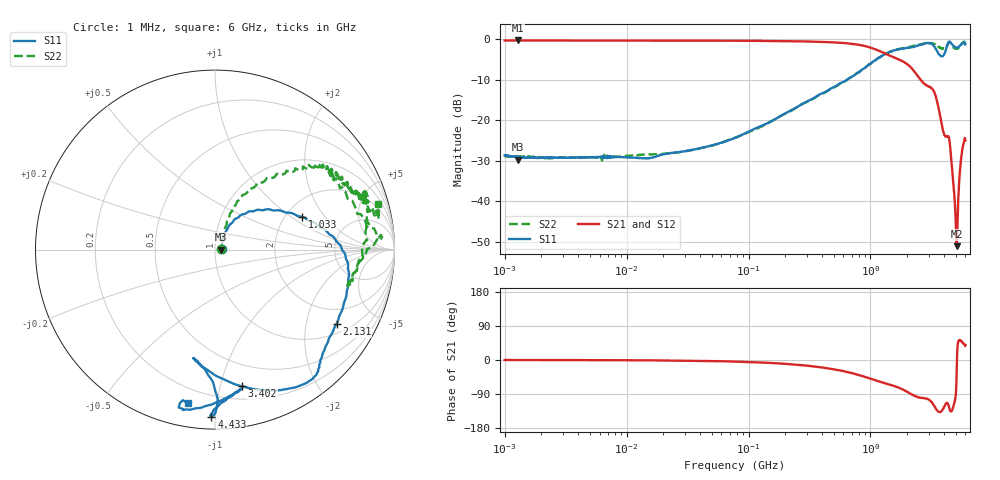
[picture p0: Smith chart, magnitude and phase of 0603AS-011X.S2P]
!s-Parameter Generated by FASTRON Sdn. Bhd.
!FASTRON P/N : 0603AS-011X
!Keysight Technologies: E5071C_MY46733604_B.14.02
!Date: Thu Nov 23 09:53:46 2023
!Version  :Rev01  Thu Nov 23 09:53:46 2023
!Data & Calibration Information:
!Freq  S11:SOLT2(ON)  S21:SOLT2(ON)  S12:SOLT2(ON)  S22:SOLT2(ON)
!PortZ  Port1:50+j0  Port2:50+j0
!When reading reference impedance value at option line is always used.
! Remarks : This data is being provided solely for informational purposes.
# Hz S dB R 50
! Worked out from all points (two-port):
!   1601 points, 1 MHz to 6 GHz, reference 50 ohm
!   highest |S21| = -0.29 dB at 1.281 MHz (marker M1); lowest = -51.1 dB at 5.105 GHz (marker M2)
!   |S21| within 3 dB of the highest: start of sweep to 1.274 GHz
!   lowest |S11| = -29.7 dB at 1.288 MHz (marker M3), VSWR 1.07, Z = 53.4 + j0.0425 ohm
!   |S11| at or under -10 dB: start of sweep to 641.8 MHz
!   |S22| runs from -30.0 to -0.5 dB; largest |S21 - S12| = 0.0099
!   S11 on the Smith chart (normalised r, x): 1 MHz: 1.08, +0.00; 1.033 GHz: 2.45, +1.22; 2.131 GHz: 1.35, -3.01; 3.402 GHz: 0.30, -1.17; 4.433 GHz: 0.07, -0.98; 6 GHz: 0.12, -0.83
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1000000  -28.66 3.2  -0.31 -0.0  -0.31 -0.1  -28.85 2.9
1281258  -28.89 3.6  -0.29 -0.1  -0.31 -0.1  -29.15 -1.2
1287650  -29.70 0.7  -0.33 0.0  -0.30 -0.0  -28.61 0.9
4277066  -29.22 4.9  -0.32 -0.3  -0.31 -0.3  -29.21 5.1
1.823719e7  -28.75 16.4  -0.32 -1.0  -0.33 -1.0  -28.36 18.0
7.757876e7  -24.37 46.8  -0.36 -4.1  -0.36 -4.1  -24.32 48.1
3.307917e8  -14.77 57.3  -0.57 -16.4  -0.57 -16.4  -14.92 66.8
6.136873e8  -10.39 44.8  -0.94 -30.1  -0.94 -30.1  -10.45 64.8
1.032581e9  -5.71 20.6  -2.20 -50.8  -2.21 -50.8  -5.66 50.8
1.414819e9  -3.22 2.8  -3.94 -64.7  -3.94 -64.7  -3.25 41.1
2.130642e9  -2.01 -31.4  -6.91 -89.0  -6.92 -88.9  -1.78 29.9
2.98045e9  -0.90 -53.5  -11.67 -104.0  -11.64 -103.9  -0.93 19.4
3.401721e9  -2.19 -78.7  -13.72 -125.7  -13.71 -125.8  -1.34 9.1
3.644712e9  -3.69 -96.3  -17.57 -137.3  -17.57 -137.4  -1.92 -8.4
3.887702e9  -4.21 -100.9  -21.87 -131.7  -21.87 -131.8  -2.28 -14.1
4.433128e9  -0.60 -91.2  -24.95 -127.3  -24.98 -127.3  -0.60 4.2
4.656967e9  -1.23 -88.5  -31.64 -132.8  -31.67 -132.8  -1.57 13.7
4.936766e9  -1.94 -80.4  -41.33 -105.1  -41.37 -105.0  -2.15 30.4
5.104645e9  -2.05 -79.4  -51.11 -10.7  -51.24 -10.9  -2.28 32.7
5.244544e9  -1.99 -80.4  -39.53 48.4  -39.59 48.5  -2.15 34.0
5.580302e9  -1.17 -93.6  -28.58 48.5  -28.58 48.6  -1.24 17.3
6e9  -1.21 -99.8  -24.97 39.2  -24.96 39.3  -0.54 15.5
